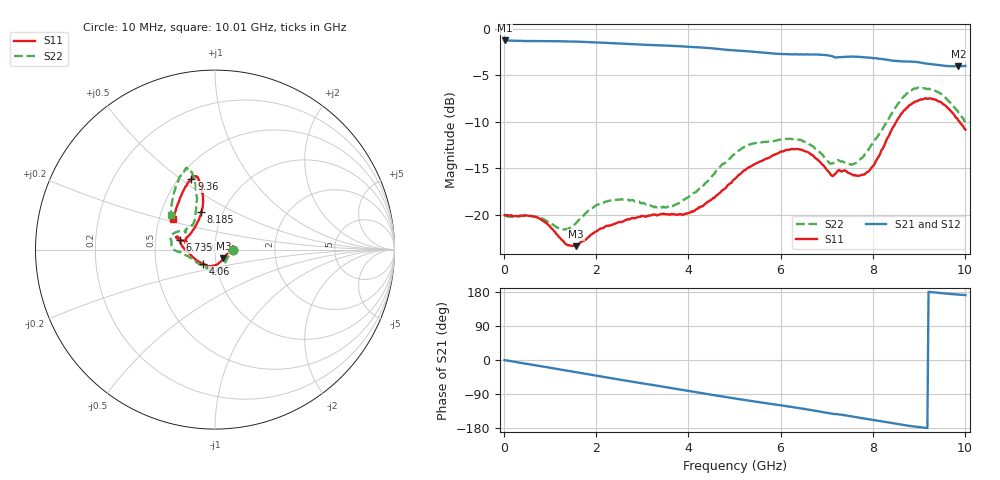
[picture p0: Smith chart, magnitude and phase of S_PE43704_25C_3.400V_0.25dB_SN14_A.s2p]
! Device ID: PE43704
! Dir: z:\PE43704\PE43704_Char_1_20130516\PE43704\AMB\3p400V\0p25dB
! Serial: 14
! Insertion: A
! Impedance: 50 ohm
! Temp: Amb
! VDD: 3.400V
! Attenuation Step: 0.25dB
! IDD: 1.141414e-01mA
#  Hz  S  RI  R  50
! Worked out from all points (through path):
!   401 points, 10 MHz to 10.01 GHz, reference 50 ohm
!   highest |S21| = -1.27 dB at 10 MHz (marker M1); lowest = -4.0 dB at 9.86 GHz (marker M2)
!   group delay of S21, straight-line fit = 53.7 ps
!   lowest |S11| = -23.4 dB at 1.56 GHz (marker M3), VSWR 1.15, Z = 54.7 - j5.36 ohm
!   |S11| at or under -10 dB: start of sweep to 8.512 GHz; 9.88 GHz to end of sweep
!   |S22| runs from -21.6 to -6.3 dB; largest |S21 - S12| = 0.0056
!   S11 on the Smith chart (normalised r, x): 10 MHz: 1.22, +0.00; 4.06 GHz: 0.86, -0.14; 6.735 GHz: 0.67, +0.08; 8.185 GHz: 0.79, +0.35; 9.36 GHz: 0.58, +0.55; 10.01 GHz: 0.59, +0.22
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1e7  0.0997 0.000151  0.8642 -0.00352  0.864 -0.00359  0.0986 0.000172
7.35e8  0.0952 0.0164  0.8275 -0.2244  0.8276 -0.2242  0.0965 0.00944
1.26e9  0.0703 -0.0195  0.7682 -0.3759  0.7683 -0.3757  0.0757 -0.0348
1.56e9  0.0472 -0.0488  0.72 -0.4552  0.7197 -0.4553  0.0569 -0.0698
1.685e9  0.0379 -0.0608  0.6969 -0.4869  0.697 -0.4867  0.0472 -0.0844
2.385e9  -0.00635 -0.089  0.5449 -0.6324  0.5452 -0.6322  -0.00144 -0.1204
3.36e9  -0.0315 -0.095  0.2958 -0.7582  0.2964 -0.7578  -0.0446 -0.1003
4.06e9  -0.0675 -0.0794  0.0999 -0.7915  0.1006 -0.7915  -0.1082 -0.0675
5.01e9  -0.1561 -0.00913  -0.1523 -0.7487  -0.152 -0.7491  -0.2132 -0.009
5.36e9  -0.1815 0.0169  -0.2354 -0.7161  -0.2356 -0.716  -0.2393 0.0152
6.085e9  -0.209 0.072  -0.3766 -0.6253  -0.3742 -0.6246  -0.2479 0.0631
6.685e9  -0.2022 0.0565  -0.4922 -0.5348  -0.4929 -0.5335  -0.213 0.0983
6.735e9  -0.1968 0.0542  -0.5014 -0.526  -0.5026 -0.5249  -0.2057 0.1004
7.11e9  -0.1569 0.0422  -0.5577 -0.4428  -0.559 -0.4439  -0.1619 0.0968
7.585e9  -0.1391 0.0846  -0.6114 -0.3566  -0.6103 -0.3559  -0.1203 0.1443
7.885e9  -0.1092 0.1303  -0.6384 -0.2857  -0.6386 -0.2887  -0.1098 0.1904
8.185e9  -0.0771 0.2076  -0.6525 -0.217  -0.6513 -0.2198  -0.1026 0.2649
8.36e9  -0.0664 0.2611  -0.6547 -0.1741  -0.654 -0.1775  -0.1017 0.3176
8.835e9  -0.0885 0.3816  -0.6618 -0.0644  -0.6583 -0.066  -0.1405 0.4428
9.36e9  -0.1317 0.3949  -0.64 0.0224  -0.641 0.0242  -0.1812 0.4265
9.86e9  -0.2108 0.2414  -0.6228 0.081  -0.621 0.0827  -0.2399 0.2607
1.001e10  -0.2321 0.1691  -0.6238 0.0945  -0.6275 0.0951  -0.2476 0.1953
